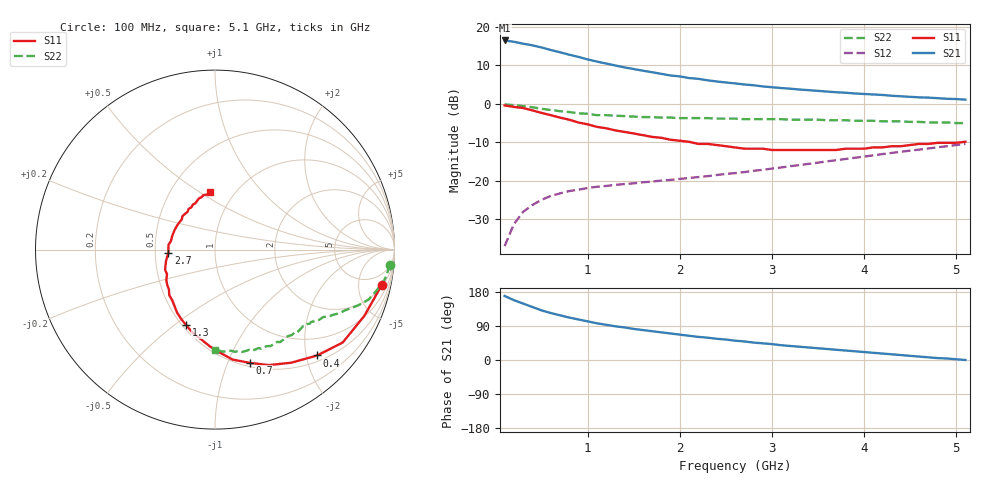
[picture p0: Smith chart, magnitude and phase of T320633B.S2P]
!AT-32063
!S AND NOISE PARAMETERS per side at Vce=2.7 V  Ic=2mA.  LAST UPDATED 11-11-96
# ghz s ma r 50
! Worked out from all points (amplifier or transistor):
!   51 points, 100 MHz to 5.1 GHz, reference 50 ohm
!   highest |S21| = 16.5 dB at 100 MHz (marker M1)
!   |S21| within 3 dB of that: start of sweep to 689.1 MHz
!   unconditionally stable (mu >= 1): 1.693 GHz to 4.514 GHz
!   at 900 MHz: K = 0.62, MSG = 17.3 dB, |S12| = -22.4 dB
!   at 2.6 GHz: K = 1.18, MAG = 9.1 dB, |S12| = -18.1 dB
!   at 5.1 GHz: K = 0.93, MSG = 5.8 dB, |S12| = -10.5 dB
!   lowest NFmin = 0.78 dB at 900 MHz
!   S11 on the Smith chart (normalised r, x): 100 MHz: 2.21, -8.97; 400 MHz: 0.61, -2.21; 700 MHz: 0.54, -1.20; 1.3 GHz: 0.52, -0.55; 2.7 GHz: 0.59, -0.02; 5.1 GHz: 0.78, +0.55
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0.1  0.95 -12.0  6.66 169.0  0.014 82.0  0.98 -5.0
0.2  0.91 -24.0  6.4 158.0  0.027 75.0  0.96 -10.0
0.3  0.88 -36.0  6.05 149.0  0.039 69.0  0.93 -14.0
0.4  0.82 -46.0  5.76 140.0  0.048 64.0  0.9 -18.0
0.5  0.76 -56.0  5.4 131.0  0.056 59.0  0.86 -21.0
0.6  0.71 -65.0  5.01 124.0  0.063 55.0  0.83 -23.0
0.7  0.66 -73.0  4.68 118.0  0.068 52.0  0.8 -25.0
0.8  0.62 -81.0  4.35 112.0  0.073 50.0  0.78 -27.0
0.9  0.57 -88.0  4.07 107.0  0.076 48.0  0.75 -29.0
1  0.54 -93.0  3.78 102.0  0.08 47.0  0.74 -30.0
1.1  0.5 -100.0  3.54 97.0  0.083 45.0  0.71 -32.0
1.3  0.45 -111.0  3.15 89.0  0.088 44.0  0.7 -34.0
1.5  0.41 -121.0  2.83 82.0  0.092 44.0  0.68 -36.0
1.8  0.36 -135.0  2.45 73.0  0.1 45.0  0.66 -39.0
1.9  0.34 -139.0  2.33 70.0  0.102 45.0  0.66 -40.0
2.2  0.3 -153.0  2.11 61.0  0.111 47.0  0.65 -44.0
2.6  0.27 -171.0  1.84 51.0  0.125 48.0  0.64 -48.0
2.7  0.26 -176.0  1.78 49.0  0.129 48.0  0.63 -50.0
3.1  0.25 164.0  1.6 39.0  0.148 49.0  0.63 -55.0
3.5  0.25 146.0  1.47 31.0  0.171 49.0  0.62 -60.0
4.3  0.28 116.0  1.27 15.0  0.229 46.0  0.59 -73.0
5.1  0.32 95.0  1.13 0.0  0.3 39.0  0.56 -90.0
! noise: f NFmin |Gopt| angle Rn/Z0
0.9  0.78  0.65  50  0.31
1.8  1.25  0.45  105  0.2
2.4  1.57  0.35  145  0.13
